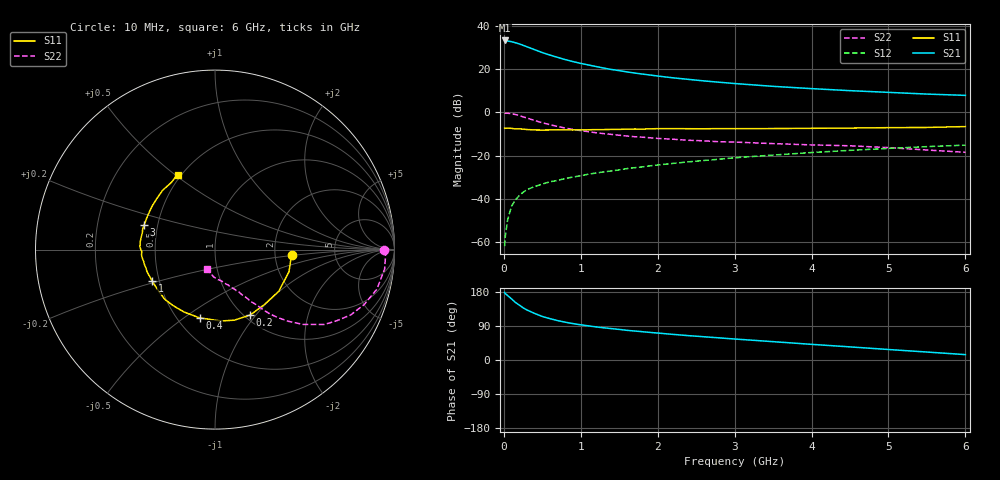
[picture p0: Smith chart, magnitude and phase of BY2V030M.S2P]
! SIEMENS Small Signal Semiconductors
! BFY420
! Si NPN RF SIEGET Grounded Emitter Transistor in MICRO-X
! VCE = 2 V  IC = 30 mA
! Common Emitter S-Parameters:  October  1996
# GHz  S  MA  R  50
!  f  S11  S21  S12  S22
! GHz  MAG  ANG  MAG  ANG  MAG  ANG  MAG  ANG
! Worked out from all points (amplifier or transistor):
!   36 points, 10 MHz to 6 GHz, reference 50 ohm
!   highest |S21| = 33.2 dB at 10 MHz (marker M1)
!   |S21| within 3 dB of that: start of sweep to 307 MHz
!   unconditionally stable (mu >= 1): start of sweep to 10.57 MHz; 1.618 GHz to end of sweep
!   at 250 MHz: K = 0.36, MSG = 34.0 dB, |S12| = -37.0 dB
!   at 1.4 GHz: K = 0.98, MSG = 23.5 dB, |S12| = -27.1 dB
!   at 6 GHz: K = 1.07, MAG = 9.9 dB, |S12| = -15.2 dB
!   S11 on the Smith chart (normalised r, x): 10 MHz: 2.48, -0.17; 200 MHz: 1.06, -0.94; 400 MHz: 0.64, -0.57; 1 GHz: 0.46, -0.19; 3 GHz: 0.42, +0.14; 6 GHz: 0.48, +0.51
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0.01  0.4278 -3.8  45.86 178.4  0.0008 115.5  0.9441 -0.3
0.02  0.4263 -6.9  45.76 175.2  0.0014 88.4  0.9511 -1.8
0.1  0.4245 -33.1  43.01 161.3  0.0067 80.2  0.9288 -13.7
0.15  0.4119 -48.0  40.61 152.0  0.0094 73.3  0.886 -20.2
0.2  0.414 -61.8  38.23 145.0  0.0118 69.9  0.8392 -25.7
0.25  0.4075 -74.8  35.42 137.8  0.0141 67.1  0.7845 -30.4
0.3  0.3992 -85.1  32.82 132.0  0.0163 65.5  0.7381 -34.4
0.4  0.39 -102.7  28.09 122.9  0.0191 62.6  0.6447 -40.3
0.5  0.3882 -116.3  24.04 114.9  0.0219 60.7  0.5725 -44.3
0.6  0.3898 -127.1  21.05 109.1  0.0247 60.9  0.5151 -47.3
0.7  0.3939 -135.4  18.6 103.9  0.0266 60.4  0.4693 -49.6
0.8  0.3902 -142.3  16.52 99.7  0.0294 59.7  0.4306 -51.3
1  0.3918 -153.2  13.51 92.9  0.0341 60.4  0.377 -53.6
1.1  0.3936 -157.7  12.43 90.0  0.037 61.2  0.3552 -55.1
1.3  0.3981 -164.8  10.54 84.9  0.0418 61.2  0.3207 -56.8
1.6  0.4078 -173.5  8.586 78.3  0.0499 60.7  0.2822 -59.9
2.2  0.419 174.1  6.264 67.6  0.0658 58.6  0.2382 -65.1
3  0.4181 160.5  4.627 55.4  0.0886 54.0  0.2047 -71.4
3.5  0.4204 152.6  3.983 48.4  0.1024 50.5  0.1885 -75.6
4.5  0.4316 138.4  3.163 34.6  0.1316 41.8  0.1679 -84.6
5.5  0.4459 123.2  2.637 21.0  0.1605 32.3  0.1341 -100.2
6  0.4672 116.5  2.461 14.2  0.1738 27.3  0.1188 -111.9
